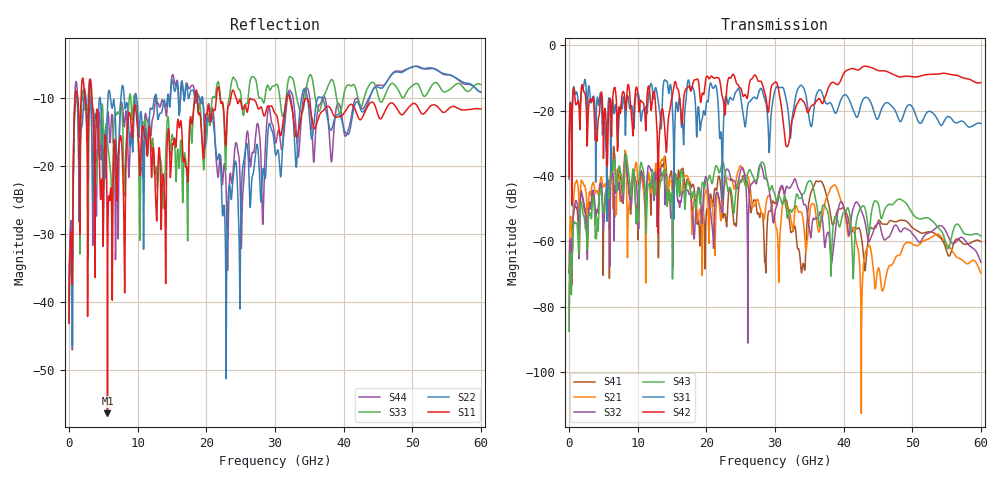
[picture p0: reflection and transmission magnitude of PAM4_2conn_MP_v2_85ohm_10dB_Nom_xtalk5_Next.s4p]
! Info: Touchstone file created by Circ.  Input file=FAB50GbE_2conn_Midplane_Examax_Topo2_v2_85ohm_10dB_Nom.circ
# Hz S RI R 50
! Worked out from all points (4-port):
!   6000 points, 10 MHz to 60 GHz, reference 50 ohm
!   strongest paths, dB at 10 MHz, 15.01 GHz, 30.01 GHz, 45.01 GHz, 60 GHz:
!     S42: -40.2, -15.9, -11.3, -7.7, -11.4
!     S31: -41.0, -17.3, -13.7, -22.5, -23.9
!     S43: -87.5, -49.4, -45.8, -48.3, -58.4
!     S32: -69.7, -53.4, -50.9, -54.3, -66.4
!     S21: -69.3, -44.4, -54.1, -68.4, -69.8
!     S41: -87.2, -40.8, -48.1, -54.1, -60.1
!   lowest |S11| = -56.4 dB at 5.6 GHz (marker M1), VSWR 1.00, Z = 49.9 + j0.0179 ohm
!   |S11| at or under -10 dB: 3.347 GHz to 18.32 GHz (14.98 GHz wide, 138 % of centre); 26.4 GHz to 31.7 GHz (5.296 GHz wide, 18.2 % of centre); 34.64 GHz to end of sweep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
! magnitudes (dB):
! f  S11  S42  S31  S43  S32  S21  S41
! 10 MHz  -43.1  -40.2  -41.0  -87.5  -69.7  -69.3  -87.2
! 1.06 GHz  -9.0  -18.1  -14.3  -54.4  -47.7  -41.5  -49.7
! 5.6 GHz  -56.4  -35.8  -24.1  -43.3  -40.9  -40.5  -41.7
! 19.18 GHz  -13.2  -17.5  -25.1  -47.9  -47.9  -51.4  -56.4
! 22.82 GHz  -17.0  -18.5  -15.7  -39.9  -38.5  -41.5  -52.9
! 42.61 GHz  -13.0  -6.9  -17.7  -49.5  -50.9  -86.9  -59.0
! 60 GHz  -11.6  -11.4  -23.9  -58.4  -66.4  -69.8  -60.1
